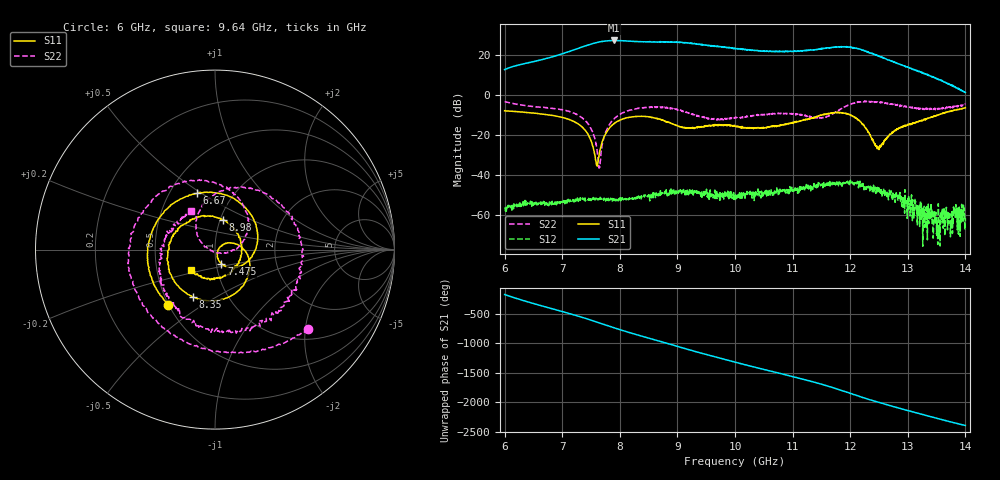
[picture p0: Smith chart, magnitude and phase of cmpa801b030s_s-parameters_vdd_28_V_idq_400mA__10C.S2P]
!Keysight Technologies,E5071C,MY46110325,B.14.03
!Date: Fri Aug 07 13:46:47 2020
!Data & Calibration Information:
!Freq	S11:SOLT2(ON)	S21:SOLT2(ON)	S12:SOLT2(ON)	S22:SOLT2(ON)
!PortZ  Port1:50+j0  Port2:50+j0
!Above PortZ is port z conversion or system Z0 setting when saving the data.
!When reading, reference impedance value at option line is always used.
# Hz S dB R 50
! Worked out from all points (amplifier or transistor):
!   1601 points, 6 GHz to 14 GHz, reference 50 ohm
!   highest |S21| = 27.3 dB at 7.905 GHz (marker M1)
!   |S21| within 3 dB of that: 7.375 GHz to 9.647 GHz (2.272 GHz wide, 26.7 % of centre)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
!   unconditionally stable (mu >= 1): start of sweep to end of sweep
!   at 7.33 GHz: K = 12.37, MAG = 24.3 dB, |S12| = -52.6 dB
!   at 10 GHz: K = 12.87, MAG = 23.8 dB, |S12| = -52.4 dB
!   at 14 GHz: K = 272.14, MAG = 4.2 dB, |S12| = -61.8 dB
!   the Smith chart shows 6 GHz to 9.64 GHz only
!   S11 on the Smith chart (normalised r, x): 6 GHz: 0.50, -0.36; 6.67 GHz: 0.68, +0.48; 7.475 GHz: 1.06, -0.17; 8.35 GHz: 0.69, -0.40; 8.98 GHz: 1.03, +0.36; 9.64 GHz: 0.75, -0.18
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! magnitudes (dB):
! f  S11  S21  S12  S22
! 6 GHz  -7.9  12.7  -56.4  -3.3
! 6.67 GHz  -9.7  17.9  -54.3  -6.2
! 7.335 GHz  -15.8  24.0  -52.5  -11.2
! 7.475 GHz  -21.2  25.3  -51.9  -15.7
! 7.59 GHz  -34.0  26.2  -52.1  -24.6
! 7.645 GHz  -29.3  26.6  -52.1  -36.4
! 7.76 GHz  -19.2  27.1  -52.4  -18.3
! 7.905 GHz  -14.2  27.3  -52.9  -11.8
! 8.35 GHz  -10.7  26.7  -51.0  -6.7
! 8.67 GHz  -12.0  26.6  -51.2  -6.1
! 8.98 GHz  -15.2  26.5  -48.4  -7.3
! 9.64 GHz  -15.1  24.7  -49.3  -11.9
! 10 GHz  -15.6  23.3  -52.4  -11.5
! 11.34 GHz  -11.7  22.6  -45.8  -11.1
! 12 GHz  -9.9  24.1  -42.9  -4.7
! 12.21 GHz  -14.7  22.5  -46.3  -3.3
! 12.48 GHz  -26.1  19.8  -48.5  -3.7
! 12.67 GHz  -20.5  17.6  -49.8  -4.2
! 13.38 GHz  -11.4  9.5  -57.2  -6.9
! 13.54 GHz  -9.9  7.9  -60.4  -6.8
! 13.84 GHz  -7.5  3.5  -55.0  -5.7
! 14 GHz  -6.4  1.3  -61.8  -4.8
